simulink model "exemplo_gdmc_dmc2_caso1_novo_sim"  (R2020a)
settings: Solver=VariableStepAuto  StartTime=0.0  StopTime=tsim  RelTol=1e-3
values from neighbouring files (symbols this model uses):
  Hc1 = H1-H2    [exemplo_gdmc_dmc2_caso1_novo.m]
  Hc2 = H1-H2    [exemplo_gdmc_dmc2_caso1_novo.m]
  Kdmc1 = Kdmc(1,:)    [exemplo_gdmc_integrador.m]    (also in exemplo_gdmc_instavel_lento.m; exemplo_gdmc_dmc2_caso1_novo.m; exemplo_gdmc_dmc2_caso3.m; gdmc_estavel.m)
  Ts = 1    [exemplo_gdmc_integrador.m]    (also in exemplo_gdmc_instavel_lento.m; exemplo_gdmc_dmc2_caso1_novo.m; exemplo_gdmc_dmc2_caso3.m; gdmc_estavel.m)
libraries: cstblocks x8, simulink x1

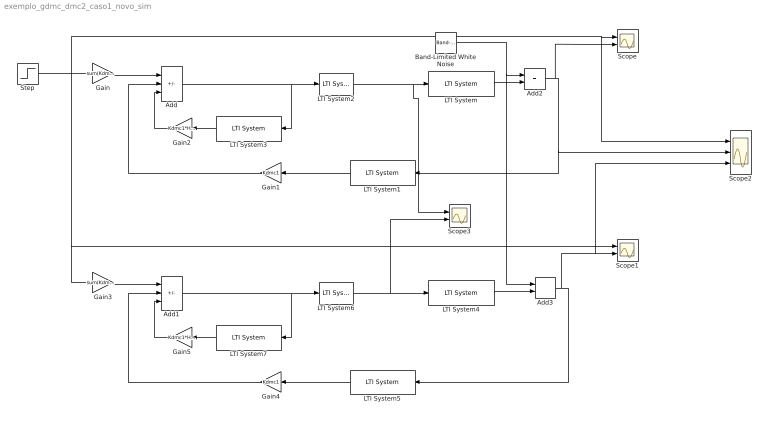
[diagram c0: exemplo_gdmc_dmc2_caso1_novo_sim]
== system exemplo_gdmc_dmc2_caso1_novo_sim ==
  Add : Sum  Inputs=+--
  Add1 : Sum  Inputs=+--
  Add2 : Sum
  Add3 : Sum
  Band-Limited White Noise : simulink/Sources/Band-Limited White Noise  Cov=[0.000001]  Ts=0.001  seed=[23341]
  Gain : Gain  Gain=sum(Kdmc1)
  Gain1 : Gain  Gain=Kdmc1  Multiplication=Matrix(K*u)
  Gain2 : Gain  Gain=Kdmc1*Hc1  Multiplication=Matrix(K*u)
  Gain3 : Gain  Gain=sum(Kdmc1)
  Gain4 : Gain  Gain=Kdmc1  Multiplication=Matrix(K*u)
  Gain5 : Gain  Gain=Kdmc1*Hc2  Multiplication=Matrix(K*u)
  LTI System : cstblocks/LTI System  sys=Gs  IC=[]
  LTI System1 : cstblocks/LTI System  sys=F1  IC=[]
  LTI System2 : cstblocks/LTI System  sys=tf([1 0],[1 -1],Ts)  IC=[]
  LTI System3 : cstblocks/LTI System  sys=gdu  IC=[]
  LTI System4 : cstblocks/LTI System  sys=Gs  IC=[]
  LTI System5 : cstblocks/LTI System  sys=F2  IC=[]
  LTI System6 : cstblocks/LTI System  sys=tf([1 0],[1 -1],Ts)  IC=[]
  LTI System7 : cstblocks/LTI System  sys=gdu  IC=[]
  Scope : Scope  NumInputPorts=2
  Scope1 : Scope  NumInputPorts=2
  Scope2 : Scope  NumInputPorts=3
  Scope3 : Scope  NumInputPorts=2
  Step : Step  Time=4*Ts  SampleTime=0
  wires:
  Gain/1 -> Add/1
  LTI System2/1 -> Scope3/1, LTI System/1
  LTI System1/1 -> Gain1/1
  Gain1/1 -> Add/2
  Gain2/1 -> Add/3
  LTI System3/1 -> Gain2/1
  Add/1 -> LTI System3/1, LTI System2/1
  Gain5/1 -> Add1/3
  Add1/1 -> LTI System7/1, LTI System6/1
  LTI System7/1 -> Gain5/1
  LTI System5/1 -> Gain4/1
  LTI System6/1 -> Scope3/2, LTI System4/1
  Gain3/1 -> Add1/1
  Step/1 -> Gain3/1, Scope1/1, Scope2/1, Scope/1, Gain/1
  Gain4/1 -> Add1/2
  LTI System/1 -> Add2/2
  LTI System4/1 -> Add3/2
  Add3/1 -> Scope2/3, Scope1/2, LTI System5/1
  Band-Limited White Noise/1 -> Add3/1, Add2/1
  Add2/1 -> Scope/2, LTI System1/1, Scope2/2
